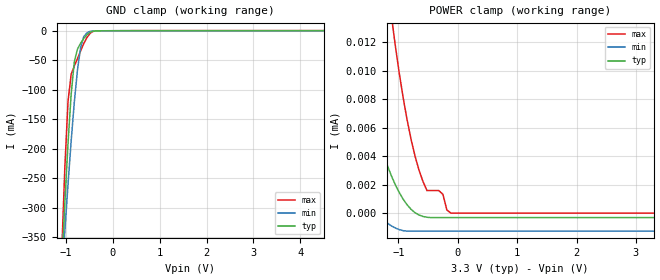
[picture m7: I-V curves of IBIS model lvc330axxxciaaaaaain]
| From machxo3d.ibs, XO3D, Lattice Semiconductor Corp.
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|   Model lvc330axxxciaaaaaain
[Model] lvc330axxxciaaaaaain
Model_type Input
Polarity   Non-Inverting
Enable   Active-High
Vinl =  0.800V
Vinh =  2.000V
C_comp   4.200pF   3.800pF   7.500pF
[Temperature Range]   25.000   0.105k   -40.000
[Voltage Range]   3.300V   3.140V   3.470V
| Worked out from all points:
|   GND clamp passes 1 mA (typ) near -0.43 V on its own axis
[GND_clamp]
|Voltage   I(typ)   I(min)   I(max)
-3.3V     -4.507A    -3.482A    -6.263A
-1.089V   -398.4mA   -420.6mA   -374.7mA
-1.022V   -290.7mA   -338.6mA   -230.6mA
-955mV    -191.3mA   -260.2mA   -120mA
-888mV    -107.5mA   -187mA     -73.65mA
-821mV    -52.97mA   -121.4mA   -59.8mA
-754mV    -31.38mA   -66.94mA   -47.42mA
-687mV    -21.14mA   -28.82mA   -34.2mA
-620mV    -13.19mA   -10.22mA   -21.96mA
-486mV    -2.621mA   -1.111mA   -4.449mA
-285mV    -80.77uA   -42.4uA    -151uA
6.6V      121.2uA    55.81uA    291.2uA
[POWER_clamp]
|Voltage   I(typ)   I(min)   I(max)
-3.3V     704.7uA    440.9uA    1.167mA
-2.596V   46.79uA    12.43uA    184.2uA
-2.328V   25.67uA    8.114uA    76.87uA
-1.792V   13.09uA    2.767uA    43.68uA
-1.39V    5.981uA    128.1nA    24.26uA
-1.122V   2.657uA    -882.9nA   13.98uA
-1.055V   2.02uA     -1.039uA   11.85uA
-854mV    586.2nA    -1.265uA   6.557uA
-653mV    -133.4nA   -1.265uA   3.018uA
-519mV    -290.3nA   -1.265uA   1.581uA
-117mV    -313.3nA   -1.265uA   0A
3.3V      -313.3nA   -1.265uA   0A
